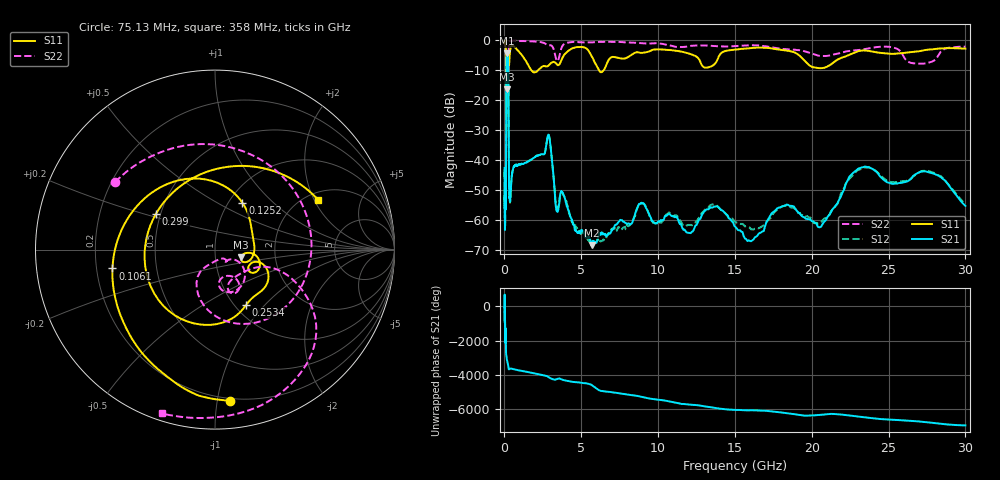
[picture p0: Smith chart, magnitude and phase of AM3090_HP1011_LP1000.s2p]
! Date/Time: Thu, Feb 28, 2019 2:05 PM
! Network Analyzer: Agilent Technologies E8364B Rev: A.07.50.67
! Sweep from 0.010 to 30.000 GHz, 1601 Points, Sweep Type: LOG
! Power Supply: 5.023 V, 0.002 A
# Hz S DB R 50
!freq MagS11 AngS11 MagS21 AngS21 MagS12 AngS12 MagS22 AngS22
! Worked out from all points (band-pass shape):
!   1601 points, 10 MHz to 30 GHz, reference 50 ohm
!   highest |S21| = -4.46 dB at 170.7 MHz (marker M1); lowest = -68.4 dB at 5.668 GHz (marker M2)
!   |S21| within 3 dB of the highest: 130.8 MHz to 243.6 MHz (112.9 MHz wide, 60.3 % of centre)
!   lowest |S11| = -16.4 dB at 158.3 MHz (marker M3), VSWR 1.36, Z = 66.8 - j5.6 ohm
!   |S11| at or under -10 dB: 124.4 MHz to 223.9 MHz (99.48 MHz wide, 57.1 % of centre); 1.743 GHz to 2.193 GHz (449.8 MHz wide, 22.9 % of centre); 6.144 GHz to 6.465 GHz (321 MHz wide, 5.09 % of centre)
!   |S22| runs from -24.6 to -0.1 dB; largest |S21 - S12| = 0.013
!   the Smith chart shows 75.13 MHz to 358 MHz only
!   S11 on the Smith chart (normalised r, x): 75.13 MHz: 0.18, -1.09; 106.1 MHz: 0.27, -0.08; 125.2 MHz: 1.16, +0.66; 253.4 MHz: 1.12, -0.79; 299 MHz: 0.47, +0.22; 358 MHz: 2.29, +2.14
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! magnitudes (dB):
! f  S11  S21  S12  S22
! 10 MHz  -0.2  -42.7  -45.7  -0.6
! 38.04 MHz  -0.4  -60.3  -59.1  -1.4
! 75.13 MHz  -1.5  -53.7  -53.9  -3.5
! 93.63 MHz  -3.0  -53.2  -54.2  -5.0
! 106.1 MHz  -4.7  -37.3  -36.6  -5.4
! 125.2 MHz  -10.4  -10.6  -10.5  -16.4
! 144.7 MHz  -13.7  -5.2  -5.2  -20.3
! 158.3 MHz  -16.4  -4.6  -4.6  -18.6
! 170.7 MHz  -13.5  -4.5  -4.4  -13.6
! 253.4 MHz  -9.0  -10.0  -10.0  -13.5
! 299 MHz  -8.3  -49.1  -49.2  -1.0
! 358 MHz  -3.9  -53.2  -54.0  -0.4
! 550.5 MHz  -2.0  -43.3  -43.1  -0.2
! 2.084 GHz  -10.6  -38.7  -38.6  -0.5
! 2.884 GHz  -8.4  -31.8  -31.7  -1.8
! 3.402 GHz  -8.0  -57.1  -56.1  -6.9
! 5.668 GHz  -5.3  -68.4  -68.4  -0.8
! 7.926 GHz  -6.0  -61.2  -62.9  -0.8
! 16.21 GHz  -2.6  -66.6  -63.3  -1.7
! 20.72 GHz  -9.3  -61.3  -60.1  -5.3
! 23.36 GHz  -3.4  -42.4  -42.8  -3.1
! 30 GHz  -2.9  -55.4  -54.8  -2.2
